PROGRAM TimeGet
//需要用到Tc2_System库和Tc2_Utilities库
VAR
	GETSYSTEMTIME: GETSYSTEMTIME;
	timeAsFileTime: T_FILETIME;
	timeAsSystemTime: TIMESTRUCT;	
	Temp1 		: T_ULARGE_INTEGER;
	Remainder: T_ULARGE_INTEGER;	//余数
	// UTC小于1ms的部分,单位ms
	ms1: LREAL;
	
	FB_LocalSystemTime:FB_LocalSystemTime;
	benable: BOOL;
	local_systemtime: Tc2_Utilities.TIMESTRUCT;
END_VAR

FB_LocalSystemTime(
	sNetID:='' , 
	bEnable:=benable , 
	dwCycle:= , 
	dwOpt:= , 
	tTimeout:= , 
	bValid=> , 
	systemTime=>local_systemtime , 
	tzID=> );
//获取UTC时间，格林尼治时间，伦敦时间，北京时间需要在这个时间上加8
GETSYSTEMTIME(
			timeLoDW=>timeAsFileTime.dwLowDateTime , 
			timeHiDW=>timeAsFileTime.dwHighDateTime );


//由于文件时间是以100ns为单位的64位无符号长整型，所以除以10000（16#2710）的余数就是小于ms的数值部分
Temp1 := UInt64Div64Ex( ULARGE_INTEGER( timeAsFileTime.dwHighDateTime, timeAsFileTime.dwLowDateTime ),
						ULARGE_INTEGER( 16#0, 16#2710 ),
						Remainder );
						
//小于1ms的时间转换成以ms为单位表示						
ms1:=UINT64_TO_LREAL(in:=ULARGE_INTEGER( Remainder.dwHighPart, Remainder.dwLowPart ))/10000.0;

END_PROGRAM
